(* Logix 5000 Rung export; software revision 16.00 *)

MODULES
   InSight_GenEth : vendor None type None code None
END_MODULES

TYPE InspectionResults_1 :   // Inspection Results from Camera
STRUCT
   InspectionResults : SINT[484];
END_STRUCT
END_TYPE

TYPE INSIGHT_OUT_1 :
STRUCT
   Control : CONTROL_OUT_1;
   UserData : SINT[488];
END_STRUCT
END_TYPE

TYPE STATUS_IN_1 :
STRUCT
   TriggerReady : BOOL;
   TriggerAck : BOOL;
   Reserved0_2 : BOOL;
   AcqError : BOOL;
   OfflineReason0 : BOOL;
   OfflineReason1 : BOOL;
   OfflineReason2 : BOOL;
   Online : BOOL;
   Reerved1_0 : BOOL;
   InspectionCompleted : BOOL;
   ResultsBufferOverrun : BOOL;
   ResultsValid : BOOL;
   CommandExecuting : BOOL;
   CommandCompleted : BOOL;
   CommandFailed : BOOL;
   Error : BOOL;
   SetUserDataAck : BOOL;
   Reserved2_1 : BOOL;
   Reserved2_2 : BOOL;
   ExposureComplete : BOOL;
   JobPass : BOOL;
   TestRunReady : BOOL;
   Reserved2_6 : BOOL;
   Reserved2_7 : BOOL;
   ExternalEventAck0 : BOOL;
   ExternalEventAck1 : BOOL;
   ExternalEventAck2 : BOOL;
   ExternalEventAck3 : BOOL;
   ExternalEventAck4 : BOOL;
   ExternalEventAck5 : BOOL;
   ExternalEventAck6 : BOOL;
   ExternalEventAck7 : BOOL;
   ErrorID : INT;
   CommandResultCode : INT;
   CurrentJobID : INT;
   AcquisitionID : INT;
   InspectionID : INT;
   InspectionResultCode : INT;
END_STRUCT
END_TYPE

TYPE CONTROL_OUT_1 :
STRUCT
   TriggerEnable : BOOL;
   Trigger : BOOL;
   BufferResultsEnable : BOOL;
   InspectionResultsAck : BOOL;
   ExecuteCommand : BOOL;
   Reserved0_5 : BOOL;
   Reserved0_6 : BOOL;
   SetOffline : BOOL;
   Reserved_Byte1 : SINT;
   SetUserData : BOOL;
   Reserved2_1 : BOOL;
   ClearError : BOOL;
   ClearExposureComplete : BOOL;
   Reserved2_4 : BOOL;
   Reserved2_5 : BOOL;
   Reserved2_6 : BOOL;
   Reserved2_7 : BOOL;
   ExternalEvent0 : BOOL;
   ExternalEvent1 : BOOL;
   ExternalEvent2 : BOOL;
   ExternalEvent3 : BOOL;
   ExternalEvent4 : BOOL;
   ExternalEvent5 : BOOL;
   ExternalEvent6 : BOOL;
   ExternalEvent7 : BOOL;
   CommandID : INT;
   Reserved_Bytes6and7 : INT;
END_STRUCT
END_TYPE

TYPE INSIGHT_IN_1 :
STRUCT
   Status : STATUS_IN_1;
   InspectionResults : InspectionResults_1;
END_STRUCT
END_TYPE

VAR_GLOBAL   (* controller tags *)
   InSight_In : INSIGHT_IN_1;
   InSight_GenEth:O : AB:ETHERNET_MODULE_DINT_496Bytes:O:0;
   InSight_Out : INSIGHT_OUT_1;
   InSight_GenEth:I : AB:ETHERNET_MODULE_DINT_500Bytes:I:0;
END_VAR

PROGRAM MainProgram

ROUTINE MainRoutine   (* ladder *)
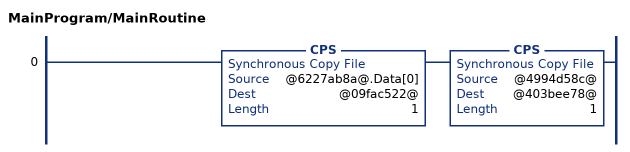
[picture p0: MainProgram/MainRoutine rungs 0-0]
   0: CPS(@6227ab8a@.Data[0],@09fac522@,1)CPS(@4994d58c@,@403bee78@,1);
END_ROUTINE
END_PROGRAM
